PROGRAM PRG_WRITE
VAR
	(* Declarations for UA_Connect *)
	fbUA_Connect			: UA_Connect;
	SessionConnectInfo		: ST_UASessionConnectInfo;
	nConnectionHdl			: DWORD;

	(* Declarations for UA_GetNamespaceIndex *)
	fbUA_GetNamespaceIndex 	: UA_GetNamespaceIndex;
	nNamespaceIndex			: UINT;

	(* Declarations for UA_NodeGetHandle *)
	fbUA_NodeGetHandle		: UA_NodeGetHandle;
	NodeID					: ST_UANodeID;
	nNodeHdl				: DWORD;

	(* Declarations for UA_Write *)
	fbUA_Write				: UA_Write;
	stIndexRange			: ARRAY [1..nMaxIndexRange] OF ST_UAIndexRange;
	nIndexRangeCount		: UINT;
	stNodeAddInfo			: ST_UANodeAdditionalInfo;
	sNodeIdentifier			: STRING(MAX_STRING_LENGTH) := 'MAIN.nNumber'; // change to node identifier
	nWriteData				: INT := 42;		// change according to the type of variable that should be written
	
	(* Declarations for UA_NodeReleaseHandle *)
	fbUA_NodeReleaseHandle	: UA_NodeReleaseHandle;

	(* Declarations for UA_Disconnect *)
	fbUA_Disconnect			: UA_Disconnect;

	(* Other declarations *)
	iState			: INT;
	bTest			: BOOL := TRUE;
	bDone			: BOOL;
	bBusy			: BOOL;
	bError			: BOOL;
	nErrorID		: DWORD;
END_VAR

CASE iState OF
0:	(* idle *)
	IF bTest THEN
		bTest	:= FALSE;
		bError	:= FALSE;
		nErrorID	:= 0;

		SessionConnectInfo.tConnectTimeout 		:= T#1M;
		SessionConnectInfo.tSessionTimeout 		:= T#1M;
		SessionConnectInfo.sApplicationName		:= '';
		SessionConnectInfo.eSecurityMode 		:= eUASecurityMsgMode_None;
		SessionConnectInfo.eSecurityPolicyUri 	:= eUASecurityPolicy_None;
		SessionConnectInfo.eTransportProfileUri := eUATransportProfileUri_UATcp;

		stNodeAddInfo.nIndexRangeCount := nIndexRangeCount;
		stNodeAddInfo.stIndexRange := stIndexRange;
		iState	:= iState + 1;
	END_IF

1:	(* open UA session *)
	fbUA_Connect(
		Execute				:= TRUE,
		ServerURL			:= sOpcUaServerUrl,
		SessionConnectInfo	:= SessionConnectInfo,
		Timeout				:= T#2M,
		ConnectionHdl		=> nConnectionHdl
	);

	IF NOT fbUA_Connect.Busy THEN
		fbUA_Connect(Execute := FALSE);

		IF NOT fbUA_Connect.Error THEN
			(* session open *)
			iState := iState + 1;
		ELSE
			bError			:= TRUE;
			nErrorID		:= fbUA_Connect.ErrorID;
			nConnectionHdl	:= 0;
			iState 			:= 0; (* idle *)
		END_IF
	END_IF


2:	(* GetNS Index *)
	fbUA_GetNamespaceIndex(
		Execute			:= TRUE,
		ConnectionHdl	:= nConnectionHdl,
		NamespaceUri	:= sNamespaceUri,
		NamespaceIndex	=> nNamespaceIndex
	);

	IF NOT fbUA_GetNamespaceIndex.Busy THEN
		fbUA_GetNamespaceIndex(Execute := FALSE);

		IF NOT fbUA_GetNamespaceIndex.Error THEN
			iState 		:= iState + 1;
		ELSE
			bError		:= TRUE;
			nErrorID	:= fbUA_GetNamespaceIndex.ErrorID;
			iState 		:= 6; (* idle *)
		END_IF
	END_IF


3:	(* Get Node Handle *)
	NodeID.eIdentifierType := eUAIdentifierType_String;
	NodeID.nNamespaceIndex := nNamespaceIndex;
	NodeID.sIdentifier	:= sNodeIdentifier;
	fbUA_NodeGetHandle(
		Execute			:= TRUE,
		ConnectionHdl	:= nConnectionHdl,
		NodeID			:= NodeID,
		NodeHdl			=> nNodeHdl
	);

	IF NOT fbUA_NodeGetHandle.Busy THEN
		fbUA_NodeGetHandle(Execute := FALSE);

		IF NOT fbUA_NodeGetHandle.Error THEN
			iState 		:= iState + 1;
		ELSE
			bError		:= TRUE;
			nErrorID	:= fbUA_NodeGetHandle.ErrorID;
			iState 		:= 6; (* idle *)
		END_IF
	END_IF


4: 	(* UA_Write *)
	fbUA_Write(
		Execute			:= TRUE,
		ConnectionHdl	:= nConnectionHdl,
		NodeHdl			:= nNodeHdl,
		stNodeAddInfo	:= stNodeAddInfo,
		cbData			:= SIZEOF(nWriteData),
		pVariable		:= ADR(nWriteData)
		);

	IF NOT fbUA_Write.Busy THEN
		fbUA_Write(
			Execute 	:= FALSE,
			pVariable	:= ADR(nWriteData));

		IF NOT fbUA_Write.Error THEN
			iState 		:= iState + 1;
		ELSE
			bError		:= TRUE;
			nErrorID	:= fbUA_Write.ErrorID;
			iState 		:= 6; (* idle *)
		END_IF
	END_IF


5:	(* Release Node Handle *)
	fbUA_NodeReleaseHandle(
		Execute			:= TRUE,
		ConnectionHdl	:= nConnectionHdl,
		NodeHdl			:= nNodeHdl
	);

	IF NOT fbUA_NodeReleaseHandle.Busy THEN
		fbUA_NodeReleaseHandle(Execute := FALSE);

		IF NOT fbUA_NodeReleaseHandle.Error THEN
			iState 		:= iState + 1;
		ELSE
			bError		:= TRUE;
			nErrorID	:= fbUA_NodeReleaseHandle.ErrorID;
			iState 		:= 6; (* idle *)
		END_IF
	END_IF


6:	(* close session *)
	fbUA_Disconnect(
		Execute			:= TRUE,
		ConnectionHdl	:= nConnectionHdl
	);

	IF NOT fbUA_Disconnect.Busy THEN
		fbUA_Disconnect(Execute := FALSE);
		bBusy := FALSE; 
		IF NOT fbUA_Disconnect.Error THEN
			(* session closed *)
			iState 		:= 0;
			IF NOT bError THEN 
				bDone 	:= TRUE;
			END_IF
		ELSE
			bError			:= TRUE;
			nErrorID		:= fbUA_Disconnect.ErrorID;
			iState 			:= 0; (* idle *)
			nConnectionHdl	:= 0;
		END_IF
	END_IF
END_CASE

END_PROGRAM
